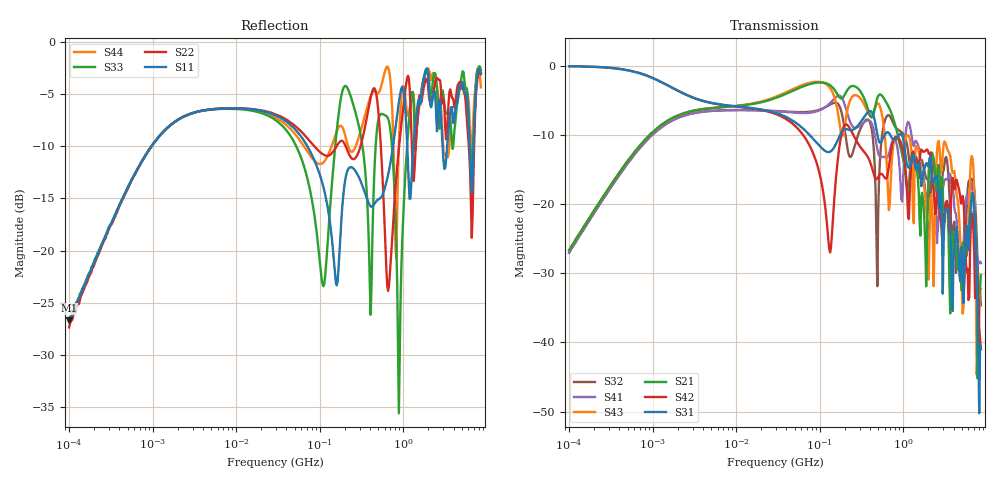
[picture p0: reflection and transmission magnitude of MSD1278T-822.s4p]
# MHz S MA R 50
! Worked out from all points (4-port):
!   498 points, 100 kHz to 8.5 GHz, reference 50 ohm
!   strongest paths, dB at 100 kHz, 1.698 MHz, 29.49 MHz, 500.7 MHz, 8.5 GHz:
!     S31: -0.1, -3.2, -6.8, -10.5, -40.9
!     S42: -0.1, -3.2, -7.0, -16.1, -41.0
!     S21: -26.7, -7.6, -4.7, -4.4, -30.3
!     S43: -26.6, -7.6, -4.5, -5.4, -32.3
!     S41: -27.0, -8.0, -6.6, -12.6, -28.6
!     S32: -27.1, -8.0, -6.5, -21.5, -34.6
!   lowest |S11| = -26.7 dB at 100 kHz (marker M1), VSWR 1.10, Z = 50.5 + j4.62 ohm
!   |S11| at or under -10 dB: 71.43 MHz to 753.1 MHz (681.7 MHz wide, 165 % of centre); 2.959 GHz to 3.353 GHz (394.2 MHz wide, 12.5 % of centre); 6.254 GHz to 6.938 GHz (683.7 MHz wide, 10.4 % of centre)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
0.1  0.04617 81.1  0.0463 82.9  0.9893 -2.7  0.04451 -97.2
     0.0463 82.9  0.04273 84.6  0.04437 -97.3  0.9906 -2.7
     0.9893 -2.7  0.04437 -97.3  0.04622 82.9  0.04666 82.8
     0.04451 -97.2  0.9906 -2.7  0.04666 82.8  0.04571 85.5
98.93298  0.2352 -63.0  0.7558 -13.9  0.2642 -81.5  0.4745 78.5
          0.7558 -13.9  0.2989 -73.5  0.4798 69.3  0.1688 -94.5
          0.2642 -81.5  0.4798 69.3  0.09317 -40.0  0.7624 -24.3
          0.4745 78.5  0.1688 -94.5  0.7624 -24.3  0.2606 -40.5
2016.336  0.6415 -178.9  0.1727 -119.3  0.1855 132.4  0.1374 160.5
          0.1727 -119.3  0.5649 -169.2  0.1384 129.5  0.2304 118.4
          0.1855 132.4  0.1384 129.5  0.7105 -167.7  0.02852 -2.1
          0.1374 160.5  0.2304 118.4  0.02852 -2.1  0.7471 -171.0
2972.863  0.3057 68.2  0.1251 26.1  0.02253 -5.9  0.1279 83.0
          0.1251 26.1  0.5178 79.5  0.1684 71.0  0.05319 -83.3
          0.02253 -5.9  0.1684 71.0  0.587 81.2  0.2303 88.1
          0.1279 83.0  0.05319 -83.3  0.2303 88.1  0.3384 37.7
5261.791  0.608 -101.6  0.05052 -172.4  0.01921 -149.3  0.04523 -91.5
          0.05052 -172.4  0.5952 -103.9  0.05297 -118.4  0.1059 155.7
          0.01921 -149.3  0.05297 -118.4  0.719 -101.8  0.01833 -102.4
          0.04523 -91.5  0.1059 155.7  0.01833 -102.4  0.5861 -101.2
6764.496  0.2249 83.7  0.06824 25.2  0.1209 39.6  0.1261 26.7
          0.06824 25.2  0.149 65.2  0.1485 41.4  0.08083 24.4
          0.1209 39.6  0.1485 41.4  0.2562 104.9  0.2122 -12.8
          0.1261 26.7  0.08083 24.4  0.2122 -12.8  0.3497 58.7
8500  0.7121 -54.4  0.03063 -18.9  0.009001 -123.3  0.03735 -152.4
      0.03063 -18.9  0.7028 -53.7  0.01852 -174.1  0.00891 -145.4
      0.009001 -123.3  0.01852 -174.1  0.7362 -55.2  0.02434 -49.2
      0.03735 -152.4  0.00891 -145.4  0.02434 -49.2  0.6077 -60.3
